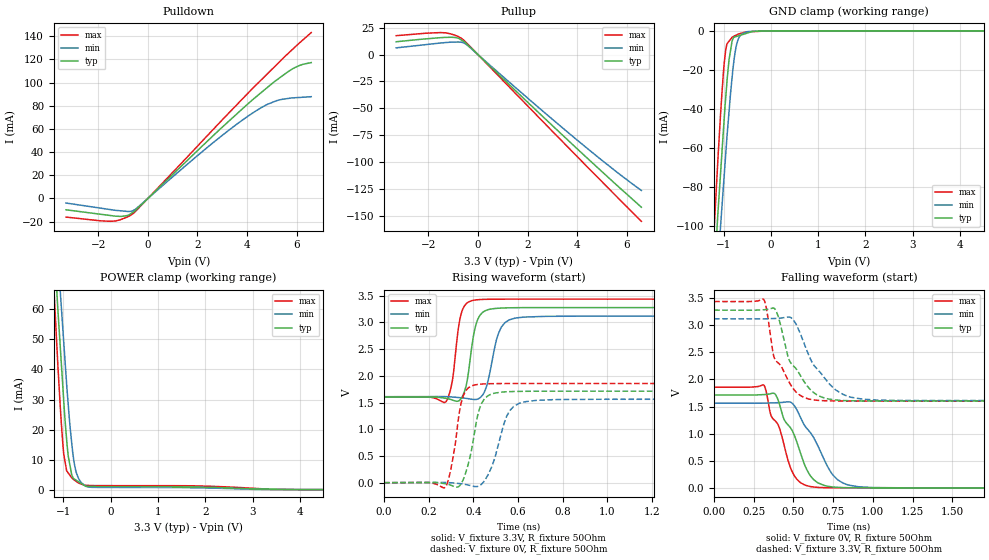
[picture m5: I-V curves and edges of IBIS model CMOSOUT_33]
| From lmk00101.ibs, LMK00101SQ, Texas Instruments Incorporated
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|   Model CMOSOUT_33
[Model]   CMOSOUT_33
Model_type   3-state
Polarity   Non-Inverting
Vmeas = 1.65
Vref = 1.65
Cref = 15pF
Rref = 50
|   typ   min   max
|   Nom   Strong   Weak
C_comp   0.4977p   0.4681p   0.5375p
|Output in High
|C_Comp high   0.4977p   0.4681p   0.5375p
|Output in low
|C_Comp low   0.9197p   0.9197p   0.9197p
|Output disabled
|C_Comp disabled   0.8920p   0.8648p   0.9197p
[Voltage Range]   3.3   3.135   3.465
[Temperature Range]   45   125   -40
[Pullup Reference]   3.3   3.135   3.465
[Pulldown Reference]   0   0   0
[Power Clamp Reference]   3.3   3.135   3.465
[GND Clamp Reference]   0   0   0
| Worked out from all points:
|   slope of the pulldown table from 0 to 0.495 V, typ, clamps not added: 48.3 ohm
|   slope of the pullup table from 0 to 0.495 V, typ, clamps not added: 45 ohm
|   GND clamp passes 1 mA (typ) near -0.48 V on its own axis
|   POWER clamp passes 1 mA (typ) near -0.23 V on its own axis
|   falling waveform, V_fixture 0V, R_fixture 50Ohm: 20-80 % time 154ps typ, 178ps min, 135ps max; typ from 1.71 V to 0 V
|   rising waveform, V_fixture 3.3V, R_fixture 50Ohm: 20-80 % time 37.3ps typ, 49ps min, 32.1ps max; typ from 1.6 V to 3.28 V
|   rising waveform, V_fixture 0V, R_fixture 50Ohm: 20-80 % time 50ps typ, 66.4ps min, 40.7ps max; typ from 0 V to 1.71 V
|   falling waveform, V_fixture 3.3V, R_fixture 50Ohm: 20-80 % time 149ps typ, 181ps min, 126ps max; typ from 3.28 V to 1.6 V
[Pulldown]
|   Voltage   I(typ)   I(min)   I(max)
-3.3V     -9.819mA   -3.964mA   -16.11mA
-1.511V   -14.76mA   -9.645mA   -19.74mA
-1.069V   -15.5mA    -10.75mA   -18.05mA
-821.6mV  -14.75mA   -11.24mA   -15.96mA
-680.8mV  -13mA      -11.04mA   -14.35mA
-479.1mV  -9.851mA   -8.933mA   -10.66mA
2.643V    54.39mA    48.36mA    59.77mA
4.407V    88.51mA    76.24mA    98.83mA
5.199V    102.3mA    84.48mA    115.6mA
5.669V    109.7mA    86.37mA    125.4mA
6.065V    114.4mA    87.14mA    133.3mA
6.59V     117.3mA    87.87mA    143.2mA
[GND Clamp]
|   Voltage   I(typ)   I(min)   I(max)
-3.3V     -1.026A    -953.5mA   -1.129A
-1.313V   -171.5mA   -189.5mA   -153.1mA
-1.123V   -95.12mA   -120.5mA   -67.71mA
-1.065V   -73.92mA   -101mA     -43.78mA
-1.003V   -51.3mA    -80.07mA   -21.65mA
-953.7mV  -34.18mA   -63.31mA   -9.728mA
-883.5mV  -14.78mA   -41.4mA    -5.306mA
-821.6mV  -5.542mA   -24.61mA   -3.377mA
-776.2mV  -3.281mA   -14.53mA   -2.71mA
-680.8mV  -2.557mA   -3.877mA   -1.611mA
-128.9mV  -106.1uA   -81.39uA   -158.9uA
6.59V     0A         0A         0A
[Pullup]
|   Voltage   I(typ)   I(min)   I(max)
-3.3V     12.01mA    6.314mA    17.68mA
-1.511V   15.83mA    10.85mA    20.57mA
-1.313V   16.08mA    11.26mA    20.33mA
-970.1mV  16.06mA    11.68mA    18.38mA
-784.5mV  15.19mA    11.78mA    16.7mA
-680.8mV  13.76mA    11.57mA    15.41mA
-516.3mV  11.39mA    10.23mA    12.25mA
-404.8mV  8.943mA    8.245mA    9.658mA
2.247V    -49.65mA   -45.31mA   -53.55mA
4.254V    -93.12mA   -84.41mA   -100.9mA
5.595V    -121.5mA   -109.3mA   -132.2mA
6.59V     -142.1mA   -126.5mA   -155.2mA
[POWER Clamp]
|   Voltage   I(typ)   I(min)   I(max)
-3.3V     701.8mA    653mA      771.4mA
-1.313V   114.3mA    126.7mA    101.8mA
-1.123V   62.1mA     79.47mA    43.86mA
-1.065V   47.86mA    66.26mA    27.92mA
-1.04V    41.79mA    60.59mA    21.79mA
-990.8mV  29.66mA    49.24mA    11.89mA
-929mV    16.61mA    35.05mA    6.26mA
-895.9mV  11.2mA     28.37mA    5.546mA
-801mV    4.192mA    12.42mA    3.637mA
-739.1mV  3.244mA    6.501mA    2.874mA
-528.3mV  1.11mA     1.213mA    1.445mA
6.59V     0A         0A         0A
[Ramp]
R_load = 50
|   typ   min   max
dV/dt_r   1.00516/3.72485e-11   0.904785/4.84964e-11   1.10021/3.20345e-11
dV/dt_f   1.02727/1.54077e-10   0.93666/1.78705e-10   1.1134/1.34607e-10
[Falling Waveform]
V_fixture = 0V
V_fixture_min = 0V
V_fixture_max = 0V
R_fixture = 50Ohm
C_fixture = 0F
|   Time   V(typ)   V(min)   V(max)
0s        1.712V     1.561V     1.856V
314ps     1.72V      1.562V     1.893V
357ps     1.737V     1.566V     1.345V
382ps     1.736V     1.568V     1.243V
442ps     1.254V     1.58V      773.5mV
502ps     993.1mV    1.528V     240.7mV
623ps     164.2mV    947.5mV    17mV
750ps     15.88mV    231.3mV    1.063mV
908ps     972.5uV    21.11mV    38.62uV
4.999ns   11.29nV    41.14nV    11.71nV
[Rising Waveform]
V_fixture = 3.3V
V_fixture_min = 3.135V
V_fixture_max = 3.465V
R_fixture = 50Ohm
C_fixture = 0F
|   Time   V(typ)   V(min)   V(max)
0s        1.601V     1.609V     1.601V
278ps     1.578V     1.61V      1.517V
305ps     1.549V     1.603V     1.876V
336ps     1.533V     1.592V     2.961V
360ps     1.695V     1.582V     3.305V
420ps     3.051V     1.565V     3.424V
459ps     3.227V     1.797V     3.431V
525ps     3.268V     2.904V     3.434V
627ps     3.276V     3.098V     3.435V
4.999ns   3.277V     3.117V     3.435V
[Rising Waveform]
V_fixture = 0V
V_fixture_min = 0V
V_fixture_max = 0V
R_fixture = 50Ohm
C_fixture = 0F
|   Time   V(typ)   V(min)   V(max)
0s        11.29nV    41.14nV    11.71nV
275ps     -20.39mV   3.609mV    -82.18mV
301ps     -48.55mV   -1.828mV   280.7mV
353ps     37.5mV     -24.36mV   1.596V
384ps     453.3mV    -50.05mV   1.791V
432ps     1.429V     -45.3mV    1.844V
484ps     1.662V     311.9mV    1.853V
562ps     1.704V     1.338V     1.855V
683ps     1.711V     1.54V      1.856V
4.999ns   1.712V     1.561V     1.856V
[Falling Waveform]
|Gnd
V_fixture = 3.3V
V_fixture_min = 3.135V
V_fixture_max = 3.465V
R_fixture = 50Ohm
C_fixture = 0F
|   Time   V(typ)   V(min)   V(max)
0s        3.277V     3.117V     3.435V
312ps     3.283V     3.116V     3.474V
331ps     3.288V     3.118V     3.283V
380ps     3.306V     3.123V     2.391V
467ps     2.406V     3.15V      1.978V
497ps     2.256V     3.104V     1.835V
631ps     1.748V     2.251V     1.62V
813ps     1.61V      1.722V     1.602V
1.029ns   1.602V     1.618V     1.601V
4.999ns   1.601V     1.609V     1.601V
